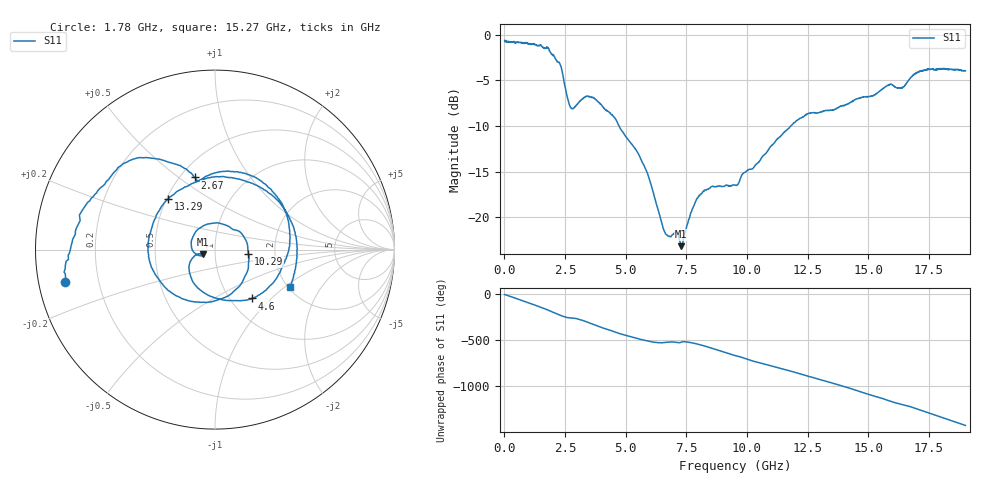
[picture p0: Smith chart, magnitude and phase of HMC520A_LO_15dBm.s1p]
! Analog Devices, Inc.
! 1 Analog Way
! Wilmington, MA 01887
! http://www.analog.com
! Date:  2021-09-07 NN
! Board Name:  EV1HMC520ALC4 Revision A with HMC520ALC4 installed
! File Description:  S-Parameters for evaluation board without connectors or board loss de-embedded
! File Generation:  Calibrated Network Analyzer
! Chip Part Number:  HMC520A
! Chip Description:  GaAs, MMIC, IQ Mixer
! Chip Frequency:  6 to 10 GHz
! Chip Package:  LCC, 3.9 x 3.9 x 0.9 mm
! Chip State:
!  Temperature:  25C
!  LO Power:  15dBm
! Note:
!  Analog Devices supplies this data as a sample of measured data at the evaluation board
!  ports for this product.  Your particular data for this product may vary.
!  Analog Devices reserves the right to change this data at anytime.
!  All lines below in this file are as is from the Network Analyzer.
!Keysight Technologies,N5245A,MY49151104,A.10.65.16
!Date: Wednesday, August 25, 2021 13:46:18
!Correction: S11(Full 2 Port(1,2))
!S1P File: Measurement: S11:
# Hz S  dB  R 50
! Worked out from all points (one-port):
!   1900 points, 10 MHz to 19 GHz, reference 50 ohm
!   lowest |S11| = -23.2 dB at 7.29 GHz (marker M1), VSWR 1.15, Z = 43.8 - j2.12 ohm
!   |S11| at or under -10 dB: 4.726 GHz to 11.81 GHz (7.085 GHz wide, 85.7 % of centre)
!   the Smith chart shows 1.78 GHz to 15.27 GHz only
!   S11 on the Smith chart (normalised r, x): 1.78 GHz: 0.08, -0.10; 2.67 GHz: 0.59, +0.57; 4.6 GHz: 1.25, -0.77; 10.29 GHz: 1.46, -0.07; 13.29 GHz: 0.51, +0.34; 15.27 GHz: 2.04, -1.10
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1e7  -0.62 -1.5
4.4e8  -0.84 -40.1
9.4e8  -0.98 -86.1
1.33e9  -1.16 -123.3
1.78e9  -1.39 -167.9
2.39e9  -4.14 124.9
2.67e9  -7.59 105.6
3.32e9  -6.81 68.4
3.79e9  -7.14 21.6
4.6e9  -9.34 -53.0
4.76e9  -10.19 -66.7
5.68e9  -13.98 -132.9
7.14e9  -21.85 -164.3
7.29e9  -23.18 -159.7
8.1e9  -17.46 169.9
9.51e9  -16.48 55.3
1.029e10  -14.52 -7.5
1.188e10  -9.81 -119.5
1.259e10  -8.58 -174.3
1.329e10  -8.30 132.7
1.426e10  -7.42 57.7
1.527e10  -6.58 -26.8
1.59e10  -5.44 -80.5
1.663e10  -5.09 -132.2
1.73e10  -3.86 168.5
1.803e10  -3.71 102.9
1.845e10  -3.79 64.6
1.9e10  -3.96 15.8
